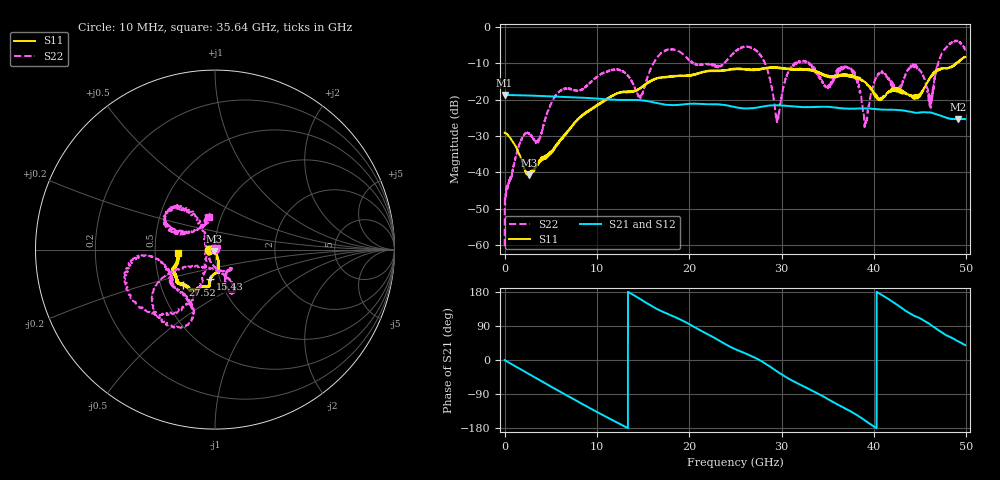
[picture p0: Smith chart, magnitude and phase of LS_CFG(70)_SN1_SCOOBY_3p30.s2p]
!Keysight Technologies,N5245B,MY58422026,A.13.80.08
!Date: Thursday, March 19, 2020 23:48:56
!Correction: S11(Full 2 Port(1,2))
!S21(Full 2 Port(1,2))
!S12(Full 2 Port(1,2))
!S22(Full 2 Port(1,2))
!S2P File: Measurements: S11, S21, S12, S22:
# Hz S DB R 50.0
!freq dBS11 angS11 dBS21 angS21 dBS12 angS12 dBS22 angS22
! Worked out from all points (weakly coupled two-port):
!   4991 points, 10 MHz to 49.91 GHz, reference 50 ohm
!   highest |S21| = -18.66 dB at 10 MHz (marker M1); lowest = -25.4 dB at 49.11 GHz (marker M2)
!   lowest |S11| = -40.8 dB at 2.63 GHz (marker M3), VSWR 1.02, Z = 49.5 - j0.779 ohm
!   |S11| at or under -10 dB: start of sweep to 48.88 GHz; 48.94958 GHz to 48.98094 GHz (31.37 MHz wide, 0.0641 % of centre)
!   |S22| runs from -60.3 to -3.7 dB; largest |S21 - S12| = 0.0011
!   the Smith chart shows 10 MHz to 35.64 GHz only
!   S11 on the Smith chart (normalised r, x): 10 MHz: 0.93, -0.01; 15.43 GHz: 0.90, -0.30; 27.52 GHz: 0.65, -0.28; 35.64 GHz: 0.66, -0.02
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1e7  -29.08 -175.5  -18.66 -0.3  -18.65 -0.3  -60.33 102.4
1.36e9  -33.67 -172.3  -18.74 -19.1  -18.73 -19.1  -34.17 -6.1
2.63e9  -40.79 -120.6  -18.84 -36.8  -18.83 -36.8  -29.39 64.2
8.33e9  -24.67 -74.0  -19.41 -114.8  -19.40 -114.8  -17.23 -59.5
1.543e10  -15.62 -98.8  -20.35 149.8  -20.35 149.9  -14.39 -150.5
1.665e10  -14.06 -99.3  -20.99 132.9  -20.98 133.0  -7.98 -146.9
1.985e10  -13.32 -105.6  -21.16 96.7  -21.15 96.8  -8.83 -108.8
2.496e10  -11.58 -122.1  -22.00 28.8  -21.98 29.0  -6.83 -172.1
2.752e10  -11.48 -132.2  -22.07 1.0  -22.06 1.3  -7.03 -125.3
2.953e10  -11.28 -140.0  -21.52 -30.3  -21.51 -30.0  -25.96 -178.0
3.094e10  -11.59 -144.8  -21.75 -51.5  -21.75 -51.3  -11.63 126.7
3.328e10  -11.84 -156.6  -22.00 -80.4  -21.99 -80.0  -10.78 156.4
3.564e10  -13.85 -175.2  -22.06 -111.8  -22.01 -111.3  -14.49 98.3
3.771e10  -13.78 172.1  -22.45 -138.9  -22.38 -139.0  -12.17 135.5
3.905e10  -15.09 169.7  -22.36 -159.7  -22.35 -159.9  -26.87 -124.5
4.032e10  -19.51 152.3  -22.59 179.6  -22.59 179.4  -13.47 -4.9
4.16e10  -17.69 106.4  -22.74 160.7  -22.77 160.7  -14.36 26.2
4.445e10  -19.16 56.2  -23.57 115.8  -23.58 116.1  -10.49 -14.9
4.614e10  -13.73 10.5  -23.50 92.9  -23.51 93.1  -21.71 -43.6
4.735e10  -11.28 9.8  -24.50 72.6  -24.51 72.8  -7.26 -83.1
4.911e10  -9.64 -12.9  -25.42 49.2  -25.44 49.3  -3.84 -43.9
4.991e10  -8.20 -13.8  -25.33 39.0  -25.35 39.0  -6.15 -28.4
